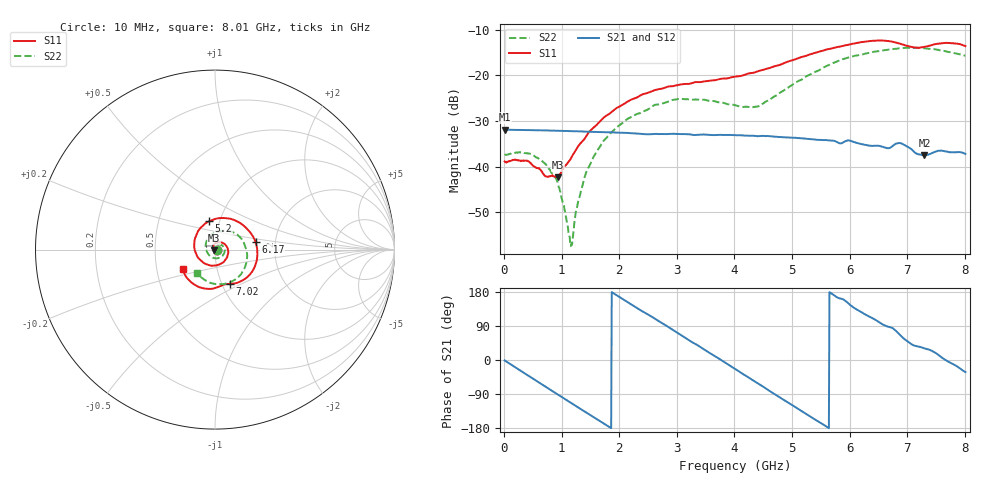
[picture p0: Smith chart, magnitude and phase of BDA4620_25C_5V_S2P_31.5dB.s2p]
!Agilent Technologies,E5071B,MY42404982,A.09.10
!Date: Wed May 06 09:05:19 2026
!Data & Calibration Information:
!Freq	S11:SOLT2(ON)	S21:SOLT2(ON)	S12:SOLT2(ON)	S22:SOLT2(ON)
# Hz S RI R 50
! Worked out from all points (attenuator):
!   801 points, 10 MHz to 8.01 GHz, reference 50 ohm
!   highest |S21| = -31.87 dB at 10 MHz (marker M1); lowest = -37.5 dB at 7.3 GHz (marker M2)
!   lowest |S11| = -42.4 dB at 930 MHz (marker M3), VSWR 1.02, Z = 49.4 - j0.443 ohm
!   |S11| at or under -10 dB: start of sweep to end of sweep
!   |S22| runs from -57.4 to -13.9 dB; largest |S21 - S12| = 0.00018
!   S11 on the Smith chart (normalised r, x): 10 MHz: 1.02, -0.00; 5.2 GHz: 0.89, +0.29; 6.17 GHz: 1.57, +0.14; 7.02 GHz: 1.09, -0.44; 8.01 GHz: 0.68, -0.16
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1e7  0.0114 -0.000684  0.0255 -0.000524  0.0255 -0.000532  0.0134 -0.000415
4.9e8  0.00741 -0.00741  0.0168 -0.0187  0.0168 -0.0187  0.0125 -0.00499
7.2e8  0.000667 -0.00779  0.00838 -0.0235  0.00837 -0.0235  0.00836 -0.00673
9.3e8  -0.00615 -0.00448  -0.00031 -0.0247  -0.000337 -0.0248  0.00364 -0.00569
1.16e9  -0.0115 0.00421  -0.00954 -0.0226  -0.00956 -0.0226  -0.00118 -0.000656
1.19e9  -0.012 0.0057  -0.0107 -0.022  -0.0107 -0.0221  -0.00159 0.00021
1.35e9  -0.0126 0.0138  -0.016 -0.0183  -0.016 -0.0183  -0.00311 0.00488
1.53e9  -0.00941 0.0242  -0.0205 -0.0126  -0.0205 -0.0126  -0.00289 0.0115
1.77e9  0.0017 0.0358  -0.0236 -0.00362  -0.0236 -0.00362  0.00122 0.0204
2.15e9  0.0316 0.041  -0.0207 0.0109  -0.0207 0.0109  0.0173 0.0289
2.68e9  0.0702 0.00763  -0.00521 0.0222  -0.00516 0.0222  0.0442 0.019
3.07e9  0.0686 -0.0403  0.00926 0.0208  0.00927 0.0208  0.055 -0.00655
4.01e9  -0.06 -0.0758  0.0203 -0.00881  0.0203 -0.00888  -0.0105 -0.0461
4.43e9  -0.1119 -0.00677  0.00958 -0.0193  0.00964 -0.0194  -0.0446 -0.0112
5.2e9  -0.0345 0.1573  -0.0152 -0.0136  -0.0152 -0.0136  -0.00343 0.0931
5.35e9  0.00827 0.1727  -0.0177 -0.00922  -0.0177 -0.00922  0.0234 0.1017
6.17e9  0.2257 0.0433  -0.0113 0.0139  -0.0113 0.0139  0.1651 0.0269
6.68e9  0.1856 -0.1484  0.000717 0.0159  0.000736 0.016  0.1692 -0.0895
7.02e9  0.084 -0.1911  0.011 0.0121  0.0111 0.0121  0.1199 -0.1609
7.3e9  0.0305 -0.2032  0.0115 0.00684  0.0115 0.00688  0.0536 -0.1909
7.65e9  -0.0821 -0.2113  0.0147 0.000386  0.0148 0.000344  -0.0323 -0.1821
8.01e9  -0.1781 -0.1103  0.0117 -0.00728  0.0117 -0.00724  -0.1025 -0.1281
